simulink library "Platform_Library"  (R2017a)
settings: Solver=VariableStepAuto  StartTime=0.0  StopTime=10.0  RelTol=1e-3
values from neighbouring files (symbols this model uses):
  m = 0    [wavespec.m]
  n = 0    [wavespec.m]
  v_req_start = 14.5    [run_master.m]
  wpts = [32.8502 121.2880    [run_master.m]
undefined symbols (not defined in the file or in its folder): course_legs, course_legsBA, distnm_legs, distnm_legsBA, ship_cargo_capacity

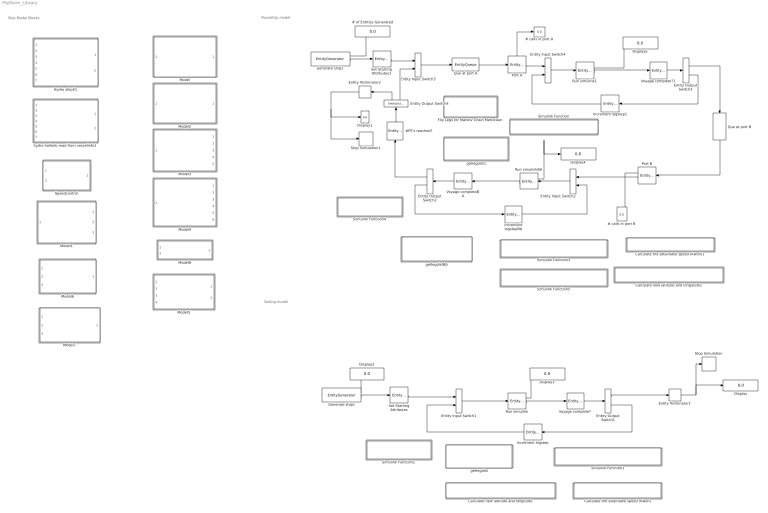
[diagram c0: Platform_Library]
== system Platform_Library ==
  note: Ship Model Blocks
  note: Roundtrip model
  note: Sailing model
  # calls in port A : Display
  # calls in port B : Display
  # of Entities Generated : Display
  #RT's reached? : EntityServer  InputPortMessageModes=m  OutputPortMessageModes=m  Capacity=1  ServiceTimeValue=0  EntryAction=|
      | %Add to the number of round trips (RTs) completed
      | entity.NumRTs=entity.NumRTs+1;
      | 
      | %Check to see if the desired number of RTs is reached
      | %If so, send entity to terminate simulation
      | entity.outputport=Completed_RT(entity.NumRTs);
  Calculate new latitude and longitude : Subsystem  TreatAsAtomicUnit=on
  Calculate new latitude and longitude1 : Subsystem  TreatAsAtomicUnit=on
  Calculate the attainable speed (Kwon) : Subsystem  TreatAsAtomicUnit=on
  Calculate the attainable speed (Kwon)1 : Subsystem  TreatAsAtomicUnit=on
  Display{,1..5} (6 alike) : Display
  Entity Input Switch{1..4} (4 alike) : EntityInputSwitch  InputPortMessageModes=m,m  OutputPortMessageModes=m
  Entity Output Switch{1..4} (4 alike) : EntityOutputSwitch  InputPortMessageModes=m  OutputPortMessageModes=m,m  SwitchingCriterion=From attribute  SwitchAttributeName=outputport
  Entity Terminator1 : EntityTerminator  InputPortMessageModes=m  NumberEntitiesArrived=on
  Entity Terminator2 : EntityTerminator  InputPortMessageModes=m  NumberEntitiesArrived=on
  Flip Legs for Markov Chain MetOcean : Subsystem  TreatAsAtomicUnit=on
  Generate ship1 : EntityGenerator  OutputPortMessageModes=n,m  TimeSource=MATLAB action  IntergenerationTimeAction=|  GenerateEntityAtSimulationStart=off  AttributeName=HsSea_S|HsdSea_S|TpSea_S|HsSwl_S|HsdSwl_S|TpSwl_S|u10_S|u10d_S|speed|outputport|legstep|legdist|leg|course|lat|lon|Hs4k|Hsd4k|Att_speed|Dist_sailed_tot|Dist_sailed_leg|numRTs|Voyage_step  AttributeInitialValue=0|0|0|0|0|0|0|0|15|1|2|1|1|1|1|1|1|1|1|0|0|1|1  NumberEntitiesDeparted=on  EntityType=Structured  EntityTypeName=ship
      | persistent count igt;
      | if isempty(count)
      |     igt=[0 inf];
      |     count=1;
      | end
      | dt=igt(count);
      | count=count+1;
  Generate ship2 : EntityGenerator  OutputPortMessageModes=n,m  TimeSource=MATLAB action  IntergenerationTimeAction=|  GenerateEntityAtSimulationStart=off  AttributeName=HsSea_S|HsdSea_S|TpSea_S|HsSwl_S|HsdSwl_S|TpSwl_S|u10_S|u10d_S|speed|outputport|legstep|legdist|leg|course|lat|lon|Hs4k|Hsd4k|Att_speed|Dist_sailed_tot|Dist_sailed_leg|NumRTs|Voyage_step|capacity  AttributeInitialValue=0|0|0|0|0|0|0|0|15|1|2|1|1|1|1|1|1|1|1|0|0|0|0|1  NumberEntitiesDeparted=on  EntityType=Structured  EntityTypeName=ship
      | persistent count igt;
      | if isempty(count)
      |     igt=[0 inf];
      |     count=1;
      | end
      | dt=igt(count);
      | count=count+1;
  Hydro shipX1 : ModelReference  ModelNameDialog=hydrodynamics.slx  SimulationMode=Normal  ModelReferenceVersion=1.29
  Increment legstep : EntityServer  InputPortMessageModes=m  OutputPortMessageModes=m  Capacity=1  ServiceTimeValue=0  EntryAction=|
      | %increment the total progress
      | entity.legstep=entity.legstep+1;
  Increment legstep1 : EntityServer  InputPortMessageModes=m  OutputPortMessageModes=m  Capacity=1  ServiceTimeValue=0  EntryAction=|
      | %increment the total progress
      | entity.legstep=entity.legstep+1;
  Increment legstepBA : EntityServer  InputPortMessageModes=m  OutputPortMessageModes=m  Capacity=1  ServiceTimeValue=0  EntryAction=|
      | %increment the total progress
      | entity.legstep=entity.legstep+1;
  Model : ModelReference  ModelNameDialog=EngRoomONE  SimulationMode=Normal  ModelReferenceVersion=1.56
  Model1 : ModelReference  ModelNameDialog=EngRoomBattery  SimulationMode=Normal  ModelReferenceVersion=1.71
  Model2 : ModelReference  ModelNameDialog=EngRoomTWO  SimulationMode=Normal  ModelReferenceVersion=1.51
  Model3 : ModelReference  ModelNameDialog=EngRoomTHREE  SimulationMode=Normal  ModelReferenceVersion=1.45
  Model4 : ModelReference  ModelNameDialog=EngRoomFOUR  SimulationMode=Normal  ModelReferenceVersion=1.44
  Model5 : ModelReference  ModelNameDialog=getLatLon  SimulationMode=Normal  ModelReferenceVersion=1.5
  Model6 : ModelReference  ModelNameDialog=Kwon_speed_loss  SimulationMode=Normal  ModelReferenceVersion=1.21
  Model7 : ModelReference  ModelNameDialog=Wind_Resistance_Model  SimulationMode=Normal  ModelReferenceVersion=1.5
  Model8 : ModelReference  ModelNameDialog=speedcontrol  SimulationMode=Normal  ModelReferenceVersion=1.22
  Port A : EntityServer  InputPortMessageModes=m  OutputPortMessageModes=n,m  Capacity=1  ServiceTimeValue=10  EntryAction=|  NumberEntitiesDeparted=on
      | %The ship is in port
      | 
      | %Run the ship model with the following modifications
      | %speed=0
      | %course=0
      | %Voyage_step: +0.5 (read as vessel being in port)
      | 
      | %run the ship model  and output the weather states (Markov Chain)
      | [HsSea_S,HsdSea_S,TpSea_S,HsSwl_S,HsdSwl_S,TpSwl_S,hsd4k,hs4k,u10_S,u10d_S]=runSim(entity.legstep, entity.course,entity.speed,entity.leg,...
      |                                                 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
  Port B : EntityServer  InputPortMessageModes=m  OutputPortMessageModes=n,m  Capacity=1  ServiceTimeValue=10  EntryAction=|  NumberEntitiesDeparted=on
      | %The ship is in port
      | 
      | %Run the ship model with the following modifications
      | %speed=0
      | %course=0
      | %Voyage_step: +0.5 (read as vessel being in port)
      | 
      | %run the ship model  and output the weather states (Markov Chain)
      | [HsSea_S,HsdSea_S,TpSea_S,HsSwl_S,HsdSwl_S,TpSwl_S,hsd4k,hs4k,u10_S,u10d_S]=runSim(entity.legstep, 0,0,entity.leg,...
      |                                                            entity.HsSwl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
  Que at port A : EntityQueue  InputPortMessageModes=m  OutputPortMessageModes=m
  Que at port B : EntityQueue  InputPortMessageModes=m  OutputPortMessageModes=m
  Run simulink : EntityServer  InputPortMessageModes=m  OutputPortMessageModes=n,m  Capacity=1  ServiceTimeValue=1  EntryAction=|  NumberEntitiesDeparted=on
      | %take the current leg, and give the vessel its course and the distance of the leg
      | [entity.course,entity.legdist]=readLeg(entity.leg);
      | 
      | %run the ship model, and output the weather states (Markov Chain)
      | [HsSea_S,HsdSea_S,TpSea_S,HsSwl_S,HsdSwl_S,TpSwl_S,hsd4k,hs4k,u10_S,u10d_S] = runSim(entity.legstep,entity.course,entity.speed,entity.leg,...
      |                                                    entity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
  Run simulink1 : EntityServer  InputPortMessageModes=m  OutputPortMessageModes=n,m  Capacity=1  ServiceTimeValue=1  EntryAction=|  NumberEntitiesDeparted=on
      | %take the current leg, and give the vessel its course and the distance of the leg
      | [entity.course,entity.legdist]=readLeg(entity.leg);
      | 
      | %run the ship model, and output the weather states (Markov Chain)
      | [HsSea_S,HsdSea_S,TpSea_S,HsSwl_S,HsdSwl_S,...
      |         TpSwl_S,hsd4k,hs4k,u10_S,u10d_S]  =  runSim(entity.legstep, entity.course,entity.speed,entity.leg,...
      |                                           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
  Run simulinkBA : EntityServer  InputPortMessageModes=m  OutputPortMessageModes=n,m  Capacity=1  ServiceTimeValue=1  EntryAction=|  NumberEntitiesDeparted=on
      | %take the current leg, and give the vessel its course and the distance of the leg
      | [entity.course,entity.legdist]=readLegBA(entity.leg); %reads from the flipped waypoints
      | 
      | %Flip leg number to collect the correct weather data for Markov Chain MetOcean
      | mc_leg=getmcleg(entity.leg);
      | 
      | %run the ship model, and output the weather states (Markov Chain)
      | [HsSea_S,HsdSea_S,TpSea_S,HsSwl_S,HsdSwl_S,...
      |        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
  Set Starting Attributes : EntityServer  InputPortMessageModes=m  OutputPortMessageModes=m  Capacity=1  ServiceTimeValue=0  EntryAction=|
      | %Read origin coordinates from waypoints
      | [lat1,lon1,v_req]=SetStart();
      | 
      | %Assign starting coordinates to entity
      | entity.lat=lat1;
      | entity.lon=lon1;
      | 
      | %Assign the intended speed
      | entity.speed=v_req;
  Set Starting Attributes1 : EntityServer  InputPortMessageModes=m  OutputPortMessageModes=m  Capacity=1  ServiceTimeValue=0  EntryAction=|
      | %Read origin coordinates from waypoints
      | [lat1,lon1,v_req,capacity]=SetStart();
      | 
      | %Assign starting coordinates to entity
      | entity.lat=lat1;
      | entity.lon=lon1;
      | 
      | %Assign the intended speed
      | entity.speed=v_req;
      | 
      | %Assign cargo capacity
      | entity.capacity=capacity;
  Simulink Function : Subsystem  TreatAsAtomicUnit=on
  Simulink Function1 : Subsystem  TreatAsAtomicUnit=on
  Simulink Function2 : Subsystem  TreatAsAtomicUnit=on
  Simulink Function3 : Subsystem  TreatAsAtomicUnit=on
  Simulink Function4 : Subsystem  TreatAsAtomicUnit=on
  Simulink Function5 : Subsystem  TreatAsAtomicUnit=on
  Speedcontrol : ModelReference  ModelNameDialog=speedcontrol.slx  SimulationMode=Normal  ModelReferenceVersion=1.22
  Stop Simulation : Stop
  Stop Simulation1 : Stop
  Voyage complete? : EntityServer  InputPortMessageModes=m  OutputPortMessageModes=m  Capacity=1  ServiceTimeValue=0  EntryAction=|
      | %Check if the entire voyage is complete
      | entity.outputport=checkComplete(entity.leg,entity.legdist,entity.Dist_sailed_leg);
      | 
      | %Check if the current Leg is complete
      | %if entity.Dist_sailed_leg>=entity.legdist
      |  %   entity.leg=entity.leg+1;%start new leg
      |  %   entity.legstep=1; %reset the counter to the new leg
      |   %  entity.Dist_sailed_leg=0; %reset the counter for distance sailed on current leg%
      | %end
  Voyage complete?1 : EntityServer  InputPortMessageModes=m  OutputPortMessageModes=m  Capacity=1  ServiceTimeValue=0  EntryAction=entity.outputport=checkComplete(entity.leg,entity.legdist,entity.Dist_sailed_leg);
  Voyage completeBA : EntityServer  InputPortMessageModes=m  OutputPortMessageModes=m  Capacity=1  ServiceTimeValue=0  EntryAction=entity.outputport=checkCompleteBA(entity.leg,entity.legdist,entity.Dist_sailed_leg);
  getlegdist : Subsystem  TreatAsAtomicUnit=on
  getlegdist1 : Subsystem  TreatAsAtomicUnit=on
  getlegdistBA : Subsystem  TreatAsAtomicUnit=on
  hydro hollenb read from vesselinfo1 : ModelReference  ModelNameDialog=hydroHollenbach  SimulationMode=Normal  ModelReferenceVersion=1.60
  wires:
  Entity Output Switch1/2 -> Increment legstep/1
  Entity Terminator1/1 -> Stop Simulation/1, Display/1
  Generate ship1/1 -> Display2/1
  Entity Output Switch1/1 -> Entity Terminator1/1
  Run simulink/2 -> Voyage complete?/1
  Set Starting Attributes/1 -> Entity Input Switch1/1
  Entity Input Switch1/1 -> Run simulink/1
  Generate ship1/2 -> Set Starting Attributes/1
  Voyage complete?/1 -> Entity Output Switch1/1
  Run simulink/1 -> Display3/1
  Increment legstep/1 -> Entity Input Switch1/2
  Que at port B/1 -> Port B/1
  Entity Input Switch2/1 -> Run simulinkBA/1
  Set Starting Attributes1/1 -> Entity Input Switch3/1
  Entity Input Switch4/1 -> Run simulink1/1
  Port B/2 -> Entity Input Switch2/1
  Run simulink1/2 -> Voyage complete?1/1
  Port B/1 -> # calls in port B/1
  Run simulinkBA/1 -> Display4/1
  Voyage complete?1/1 -> Entity Output Switch3/1
  Run simulink1/1 -> Display5/1
  Entity Terminator2/1 -> Stop Simulation1/1, Display1/1
  Increment legstepBA/1 -> Entity Input Switch2/2
  Entity Output Switch3/1 -> Que at port B/1
  #RT's reached?/1 -> Entity Output Switch4/1
  Port A/1 -> # calls in port A/1
  Generate ship2/1 -> # of Entities Generated/1
  Entity Output Switch2/1 -> #RT's reached?/1
  Entity Output Switch4/2 -> Entity Input Switch3/2
  Run simulinkBA/2 -> Voyage completeBA/1
  Entity Output Switch4/1 -> Entity Terminator2/1
  Entity Output Switch3/2 -> Increment legstep1/1
  Increment legstep1/1 -> Entity Input Switch4/2
  Voyage completeBA/1 -> Entity Output Switch2/1
  Que at port A/1 -> Port A/1
  Generate ship2/2 -> Set Starting Attributes1/1
  Entity Output Switch2/2 -> Increment legstepBA/1
  Entity Input Switch3/1 -> Que at port A/1
  Port A/2 -> Entity Input Switch4/1

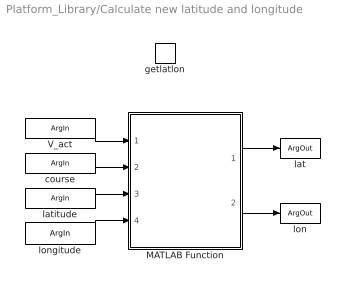
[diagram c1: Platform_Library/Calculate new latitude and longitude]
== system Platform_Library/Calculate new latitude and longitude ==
  getlatlon : TriggerPort  TriggerType=function-call  IsSimulinkFunction=on  FunctionName=getlatlon  VariantControl=Variant
  MATLAB Function : MATLAB Function  TreatAsAtomicUnit=on
  V_act : ArgIn  DisableCoverage=on  ArgumentName=V_act
  latitude : ArgIn  Port=2  ArgumentName=latitude
  longitude : ArgIn  Port=3  ArgumentName=longitude
  course : ArgIn  Port=4  ArgumentName=course
  lat : ArgOut  DisableCoverage=on  ArgumentName=lat
  lon : ArgOut  Port=2  ArgumentName=lon
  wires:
  V_act/1 -> MATLAB Function/1(V_act)
  MATLAB Function/1(lat_new) -> lat/1
  course/1 -> MATLAB Function/2(Course)
  latitude/1 -> MATLAB Function/3(Lat)
  longitude/1 -> MATLAB Function/4(Lon)
  MATLAB Function/2(lon_new) -> lon/1

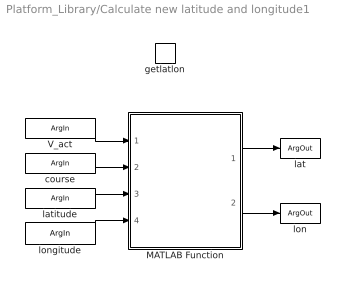
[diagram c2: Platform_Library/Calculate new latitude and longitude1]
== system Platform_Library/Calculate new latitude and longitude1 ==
  getlatlon : TriggerPort  TriggerType=function-call  IsSimulinkFunction=on  FunctionName=getlatlon  VariantControl=Variant
  MATLAB Function : MATLAB Function  TreatAsAtomicUnit=on
  V_act : ArgIn  DisableCoverage=on  ArgumentName=V_act
  latitude : ArgIn  Port=2  ArgumentName=latitude
  longitude : ArgIn  Port=3  ArgumentName=longitude
  course : ArgIn  Port=4  ArgumentName=course
  lat : ArgOut  DisableCoverage=on  ArgumentName=lat
  lon : ArgOut  Port=2  ArgumentName=lon
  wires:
  V_act/1 -> MATLAB Function/1(V_act)
  MATLAB Function/1(lat_new) -> lat/1
  course/1 -> MATLAB Function/2(Course)
  latitude/1 -> MATLAB Function/3(Lat)
  longitude/1 -> MATLAB Function/4(Lon)
  MATLAB Function/2(lon_new) -> lon/1

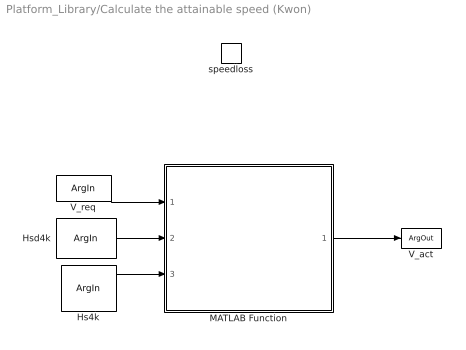
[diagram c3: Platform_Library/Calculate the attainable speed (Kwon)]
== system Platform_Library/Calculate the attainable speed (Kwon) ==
  speedloss : TriggerPort  TriggerType=function-call  IsSimulinkFunction=on  FunctionName=speedloss  VariantControl=Variant
  MATLAB Function : MATLAB Function  TreatAsAtomicUnit=on
  V_req : ArgIn  DisableCoverage=on  ArgumentName=V_req
  Hsd4k : ArgIn  Port=2  ArgumentName=Hsd4k
  Hs4k : ArgIn  Port=3  ArgumentName=Hs4k
  V_act : ArgOut  DisableCoverage=on  ArgumentName=V_act
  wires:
  MATLAB Function/1(V_act) -> V_act/1
  Hs4k/1 -> MATLAB Function/3(Hs)
  Hsd4k/1 -> MATLAB Function/2(rel_heading)
  V_req/1 -> MATLAB Function/1(V_req)

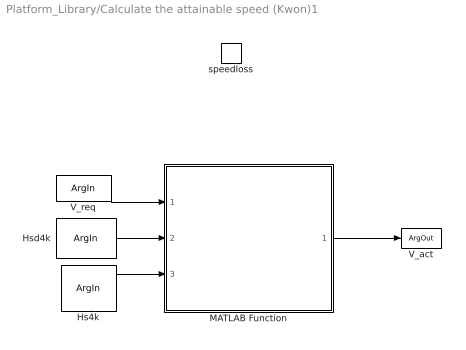
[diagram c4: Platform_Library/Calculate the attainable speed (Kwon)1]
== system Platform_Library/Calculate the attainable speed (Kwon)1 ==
  speedloss : TriggerPort  TriggerType=function-call  IsSimulinkFunction=on  FunctionName=speedloss  VariantControl=Variant
  MATLAB Function : MATLAB Function  TreatAsAtomicUnit=on
  V_req : ArgIn  DisableCoverage=on  ArgumentName=V_req
  Hsd4k : ArgIn  Port=2  ArgumentName=Hsd4k
  Hs4k : ArgIn  Port=3  ArgumentName=Hs4k
  V_act : ArgOut  DisableCoverage=on  ArgumentName=V_act
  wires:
  MATLAB Function/1(V_act) -> V_act/1
  Hs4k/1 -> MATLAB Function/3(Hs)
  Hsd4k/1 -> MATLAB Function/2(rel_heading)
  V_req/1 -> MATLAB Function/1(V_req)

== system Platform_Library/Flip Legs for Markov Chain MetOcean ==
  getmcleg : TriggerPort  TriggerType=function-call  IsSimulinkFunction=on  FunctionName=getmcleg  VariantControl=Variant
  MATLAB Function : MATLAB Function  TreatAsAtomicUnit=on
  leg : ArgIn  DisableCoverage=on  ArgumentName=leg
  mc_leg : ArgOut  DisableCoverage=on  ArgumentName=mc_leg
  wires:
  leg/1 -> MATLAB Function/1(leg)
  MATLAB Function/1(mc_leg) -> mc_leg/1

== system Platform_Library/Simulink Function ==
  Completed_RT : TriggerPort  TriggerType=function-call  IsSimulinkFunction=on  FunctionName=Completed_RT  VariantControl=Variant
  MATLAB Function : MATLAB Function  TreatAsAtomicUnit=on
  numRTs : ArgIn  DisableCoverage=on  ArgumentName=numRTs
  outputport : ArgOut  DisableCoverage=on  ArgumentName=outputport
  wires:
  numRTs/1 -> MATLAB Function/1(NumRTs)
  MATLAB Function/1(outport) -> outputport/1

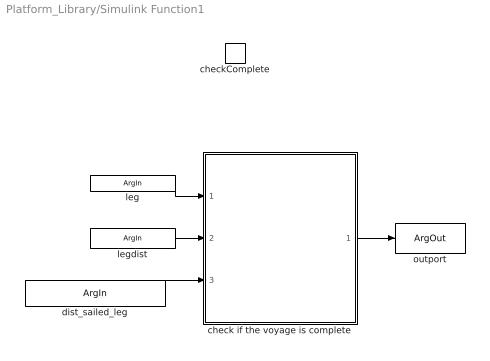
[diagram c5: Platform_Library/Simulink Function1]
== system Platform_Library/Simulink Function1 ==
  checkComplete : TriggerPort  TriggerType=function-call  IsSimulinkFunction=on  FunctionName=checkComplete  VariantControl=Variant
  check if the voyage is complete : MATLAB Function  TreatAsAtomicUnit=on
  leg : ArgIn  DisableCoverage=on  ArgumentName=leg
  legdist : ArgIn  Port=2  ArgumentName=legdist
  dist_sailed_leg : ArgIn  Port=3  ArgumentName=dist_sailed_leg
  outport : ArgOut  DisableCoverage=on  ArgumentName=outport
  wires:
  leg/1 -> check if the voyage is complete/1(leg)
  check if the voyage is complete/1(outport) -> outport/1
  dist_sailed_leg/1 -> check if the voyage is complete/3(dist_sailed_leg)
  legdist/1 -> check if the voyage is complete/2(legdist)

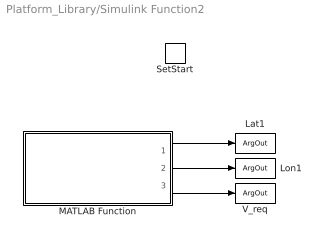
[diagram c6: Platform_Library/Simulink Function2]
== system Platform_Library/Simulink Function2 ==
  SetStart : TriggerPort  TriggerType=function-call  IsSimulinkFunction=on  FunctionName=SetStart  VariantControl=Variant
  MATLAB Function : MATLAB Function  TreatAsAtomicUnit=on
  Lat1 : ArgOut  DisableCoverage=on  ArgumentName=Lat1
  Lon1 : ArgOut  Port=2  ArgumentName=Lon1
  V_req : ArgOut  Port=3  ArgumentName=V_req
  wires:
  MATLAB Function/2(Lon1) -> Lon1/1
  MATLAB Function/1(Lat1) -> Lat1/1
  MATLAB Function/3(v_req) -> V_req/1

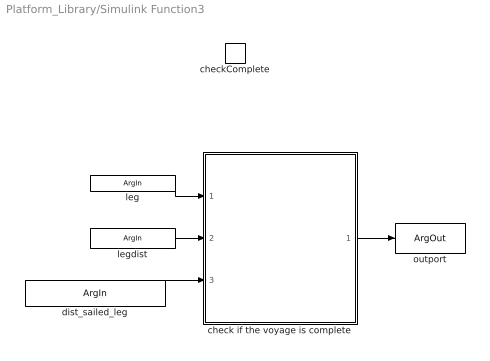
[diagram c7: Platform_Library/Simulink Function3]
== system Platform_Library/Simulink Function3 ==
  checkComplete : TriggerPort  TriggerType=function-call  IsSimulinkFunction=on  FunctionName=checkComplete  VariantControl=Variant
  check if the voyage is complete : MATLAB Function  TreatAsAtomicUnit=on
  leg : ArgIn  DisableCoverage=on  ArgumentName=leg
  legdist : ArgIn  Port=2  ArgumentName=legdist
  dist_sailed_leg : ArgIn  Port=3  ArgumentName=dist_sailed_leg
  outport : ArgOut  DisableCoverage=on  ArgumentName=outport
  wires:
  leg/1 -> check if the voyage is complete/1(leg)
  check if the voyage is complete/1(outport) -> outport/1
  dist_sailed_leg/1 -> check if the voyage is complete/3(dist_sailed_leg)
  legdist/1 -> check if the voyage is complete/2(legdist)

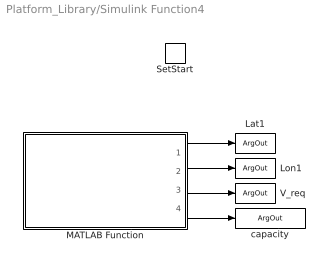
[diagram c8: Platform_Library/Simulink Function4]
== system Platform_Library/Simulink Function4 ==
  SetStart : TriggerPort  TriggerType=function-call  IsSimulinkFunction=on  FunctionName=SetStart  VariantControl=Variant
  MATLAB Function : MATLAB Function  TreatAsAtomicUnit=on
  Lat1 : ArgOut  DisableCoverage=on  ArgumentName=Lat1
  Lon1 : ArgOut  Port=2  ArgumentName=Lon1
  V_req : ArgOut  Port=3  ArgumentName=V_req
  capacity : ArgOut  Port=4  ArgumentName=capacity
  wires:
  MATLAB Function/2(Lon1) -> Lon1/1
  MATLAB Function/1(Lat1) -> Lat1/1
  MATLAB Function/3(v_req) -> V_req/1
  MATLAB Function/4(capacity) -> capacity/1

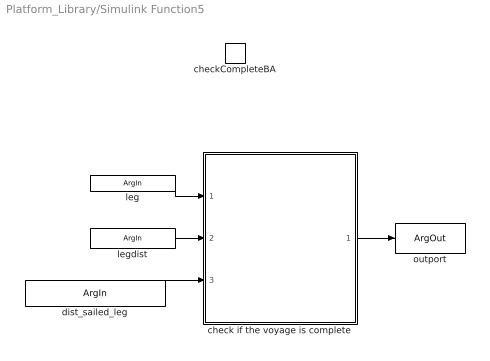
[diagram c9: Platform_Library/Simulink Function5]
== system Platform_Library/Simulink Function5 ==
  checkCompleteBA : TriggerPort  TriggerType=function-call  IsSimulinkFunction=on  FunctionName=checkCompleteBA  VariantControl=Variant
  check if the voyage is complete : MATLAB Function  TreatAsAtomicUnit=on
  leg : ArgIn  DisableCoverage=on  ArgumentName=leg
  legdist : ArgIn  Port=2  ArgumentName=legdist
  dist_sailed_leg : ArgIn  Port=3  ArgumentName=dist_sailed_leg
  outport : ArgOut  DisableCoverage=on  ArgumentName=outport
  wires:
  leg/1 -> check if the voyage is complete/1(leg)
  check if the voyage is complete/1(outport) -> outport/1
  dist_sailed_leg/1 -> check if the voyage is complete/3(dist_sailed_leg)
  legdist/1 -> check if the voyage is complete/2(legdist)

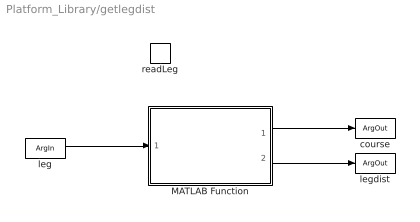
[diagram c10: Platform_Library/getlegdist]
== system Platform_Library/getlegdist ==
  readLeg : TriggerPort  TriggerType=function-call  IsSimulinkFunction=on  FunctionName=readLeg  VariantControl=Variant
  MATLAB Function : MATLAB Function  TreatAsAtomicUnit=on
  leg : ArgIn  DisableCoverage=on  ArgumentName=leg
  course : ArgOut  DisableCoverage=on  ArgumentName=course
  legdist : ArgOut  DisableCoverage=on  Port=2  ArgumentName=legdist
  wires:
  leg/1 -> MATLAB Function/1(leg)
  MATLAB Function/1(course) -> course/1
  MATLAB Function/2(legdist) -> legdist/1

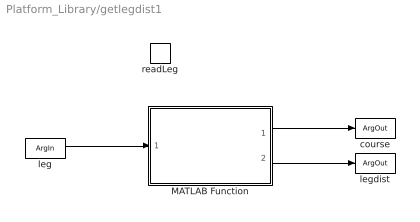
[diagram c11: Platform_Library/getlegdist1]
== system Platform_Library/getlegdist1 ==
  readLeg : TriggerPort  TriggerType=function-call  IsSimulinkFunction=on  FunctionName=readLeg  VariantControl=Variant
  MATLAB Function : MATLAB Function  TreatAsAtomicUnit=on
  leg : ArgIn  DisableCoverage=on  ArgumentName=leg
  course : ArgOut  DisableCoverage=on  ArgumentName=course
  legdist : ArgOut  DisableCoverage=on  Port=2  ArgumentName=legdist
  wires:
  leg/1 -> MATLAB Function/1(leg)
  MATLAB Function/1(course) -> course/1
  MATLAB Function/2(legdist) -> legdist/1

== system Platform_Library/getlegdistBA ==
  readLegBA : TriggerPort  TriggerType=function-call  IsSimulinkFunction=on  FunctionName=readLegBA  VariantControl=Variant
  MATLAB Function : MATLAB Function  TreatAsAtomicUnit=on
  leg : ArgIn  DisableCoverage=on  ArgumentName=leg
  course : ArgOut  DisableCoverage=on  ArgumentName=course
  legdist : ArgOut  DisableCoverage=on  Port=2  ArgumentName=legdist
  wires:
  leg/1 -> MATLAB Function/1(leg)
  MATLAB Function/1(course) -> course/1
  MATLAB Function/2(legdist) -> legdist/1

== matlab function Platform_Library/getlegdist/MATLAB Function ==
function [course,legdist] = fcn(leg,distnm_legs,course_legs)
%take in the current leg that the vessel is on, and give the distance for
%that leg, and the course
course=course_legs(leg);
legdist=distnm_legs(leg);
    
end

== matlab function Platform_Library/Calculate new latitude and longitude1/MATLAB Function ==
function [lat_new, lon_new] = New_Lat_Lon(V_act,Course,Lat,Lon)

coder.extrinsic('nm2deg')
coder.extrinsic('reckon')
time=1; % one hour time steps

lat_new=0; %preallocate
lon_new=0; %preallocate


distance=V_act*time; %distance sailed [nm]
arc_length=nm2deg(distance); %distance sailed [deg]

[lat_new, lon_new]=reckon(Lat,Lon,arc_length,Course); %new lat and lon


end

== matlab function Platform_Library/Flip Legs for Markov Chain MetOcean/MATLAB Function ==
function mc_leg = getMCleg(leg,distnm_legsBA)

%Flip the leg number to collect the correct weather data for MetOcean
%Markov Chains

num_legs=size(distnm_legsBA,1); %get the total number of legs
legs=(1:1:num_legs);
flip_legs=flip(legs);
mc_leg=flip_legs(leg);
end

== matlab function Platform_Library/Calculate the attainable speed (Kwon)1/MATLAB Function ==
function V_act = speedloss_Kwon(V_req,rel_heading,Hs, num)
coder.extrinsic('wrapTo180')
%Use Kwons method to estimate the speed loss due to added resistance

%pre allocate values
V_act=0;
V_2=0; %pre allocate the new speed
Bn=0;
Volume_deplacement=0;
C_u=0;
C_beta=0;
C_form=0;
heading_rel=0;

V_1=V_req*0.5144; %Convert the required speed (set speed) from kts to m/s
heading_rel=abs(wrapTo180(rel_heading)); %convert to 0-180 degrees
Volume_deplacement=num(54); %[m^3]
L=num(3); %Use Lwl
C_B=num(8); %block Coefficient



%calculate the current Froude Number
F_n=V_1/((9.81*L)^0.5);

%Get Beaufort scale number from waveheight
if Hs<0.2
    Bn=1;
elseif Hs>=0.2 && Hs<0.5
    Bn=2;
elseif Hs>=0.5 && Hs<1
    Bn=3;
elseif Hs>=1 && Hs<2
    Bn=4;
elseif Hs>2 && Hs<3
    Bn=5;
elseif Hs>3 && Hs<4
    Bn=6;
elseif Hs>4 %&& Hs<5.5
    Bn=7;
else
    disp('Bn is too high for Kwons method')
end
    

%calculate speed reduction coefficient
if C_B>=0.55 && C_B<0.575
    C_u=1.7-(1.4*F_n)-(7.4*(F_n^2));
elseif C_B>=0.575 && C_B<0.625
    C_u=2.2-(2.5*F_n)-(9.7*(F_n^2));
elseif C_B>=0.625 && C_B<0.675
    C_u=2.6-(3.7*F_n)-(11.6*(F_n^2));
elseif C_B>=0.675 && C_B<0.725
    C_u=3.1-(5.3*F_n)-(12.4*(F_n^2));
elseif C_B>=0.725 && C_B<0.775
    C_u=2.4-(10.6*F_n)-(9.5*(F_n^2));
elseif C_B>=0.775 && C_B<0.825
    C_u=2.6-(13.1*F_n)-(15.1*(F_n^2));
else %C_B>=0.825
    C_u=3.1-(18.7*F_n)+(28*(F_n^2));
end

%calculate direction reduction coefficient
if heading_rel>=0 && heading_rel<30 %head sea
    C_beta=1;
elseif heading_rel>=30 && heading_rel<60 %Bow sea
    C_beta=(1.7-0.03*((Bn-4)^2))/2;
elseif heading_rel>=60 && heading_rel<150 %Beam sea
    C_beta=(0.9-0.06*((Bn-6)^2))/2;
else %heading_rel>=150 && heading_rel<180 %Following sea
    C_beta=(0.4-0.03*((Bn-8)^2))/2;
end

%calculate the ship form coefficient
%valid for all ships, exept container ships, in loaded condition
%C_form=(0.5*Bn)+((Bn^(6.5))/((2.7*(Volume_deplacement^(2/3)))));

%valid for container ships in normal condition
C_form=(0.7*Bn)+((Bn^(6.5))/((22*(Volume_deplacement^(2/3)))));

%percentage loss calculated
%percentage_loss=((V_1-V_2)/V_1)*100;





%calculate deltaV/V1*100%
%Delta_V_overV=C_beta*C_u*C_form;
%coefficient=C_form*C_beta*C_u
%calculate actual ship speed in the selected weather [m/s]
% V_2=V_1-((Delta_V_overV)*(V_1/100))
V_2=V_1-((C_beta*C_u*C_form)*(V_1/100));

%calculate the absolute speed loss [m/s]
%delta_V=V_1-V_2



%if the speed loss found is negative, set the speed to the original speed
% This means that the approximate method did not work in this case
% if V_2>=V_1
%     V_2=V_1; 
%     disp('Approximate method not valid')
%     
% end

V_act=V_2/0.5144; % The actual attainable speed in kts
end


% %function V_act = speedloss_Kwon(V_req,rel_heading,Hs, num)
% %Use Kwons method to estimate the speed loss due to added resistance
% 
% V_1=V_req*0.5144; %Convert the required speed (set speed) from kts to m/s
% heading_rel=rel_heading;
% Volume_deplacement=num(54); %[m^3]
% L=num(3); %Use Lwl
% C_B=num(8); %block Coefficient
% 
% 
% %calculate the current Froude Number
% F_n=V_1/((9.81*L)^0.5);
% 
% %Get Beaufort scale number from waveheight
% if Hs<0.2
%     Bn=1;
% elseif Hs>=0.2 && Hs<0.5
%     Bn=2;
% elseif Hs>=0.5 && Hs<1
%     Bn=3;
% elseif Hs>=1 && Hs<2
%     Bn=4;
% elseif Hs>2 && Hs<3
%     Bn=5;
% elseif Hs>3 && Hs<4
%     Bn=6;
% elseif Hs>4 && Hs<5.5
%     Bn=7;
% else
%     disp('Bn is too high for Kwons method')
% end
%     
% 
% %calculate speed reduction coefficient
% if C_B>=0.55 && C_B<0.575
%     C_u=1.7-(1.4*F_n)-(7.4*(F_n^2));
% elseif C_B>=0.575 && C_B<0.625
%     C_u=2.2-(2.5*F_n)-(9.7*(F_n^2));
% elseif C_B>=0.625 && C_B<0.675
%     C_u=2.6-(3.7*F_n)-(11.6*(F_n^2));
% elseif C_B>=0.675 && C_B<0.725
%     C_u=3.1-(5.3*F_n)-(12.4*(F_n^2));
% elseif C_B>=0.725 && C_B<0.775
%     C_u=2.4-(10.6*F_n)-(9.5*(F_n^2));
% elseif C_B>=0.775 && C_B<0.825
%     C_u=2.6-(13.1*F_n)-(15.1*(F_n^2));
% elseif C_B>=0.825
%     C_u=3.1-(18.7*F_n)+(28*(F_n^2));
% end
% 
% %calculate direction reduction coefficient
% if heading_rel>=0 && heading_rel<30 %head sea
%     C_beta=1;
% elseif heading_rel>=30 && heading_rel<60 %Bow sea
%     C_beta=(1.7-0.03*((Bn-4)^2))/2;
% elseif heading_rel>=60 && heading_rel<150 %Beam sea
%     C_beta=(0.9-0.06*((Bn-6)^2))/2;
% elseif heading_rel>=150 && heading_rel<180 %Following sea
%     C_beta=(0.4-0.03*((Bn-8)^2))/2;
% end
% 
% %calculate the ship form coefficient
% %valid for all ships, exept container ships, in loaded condition
% C_form=(0.5*Bn)+((Bn^(6.5))/((2.7*(Volume_deplacement^(2/3)))));
% 
% %calculate deltaV/V1*100%
% %Delta_V_overV=C_beta*C_u*C_form;
% 
% %calculate actual ship speed in the selected weather [m/s]
% % V_2=V_1-((Delta_V_overV)*(V_1/100))
% V_2=V_1-((C_beta*C_u*C_form)*(V_1/100));
% 
% %calculate the absolute speed loss [m/s]
% %delta_V=V_1-V_2
% 
% %percentage loss calculated
% %percentage_loss=((V_1-V_2)/V_1)*100;
% 
% %if the speed loss found is negative, set the speed to the original speed
% % This means that the approximate method did not work in this case
% if V_2>=V_1
%     V_2=V_1; 
%     disp('Approximate method not valid')
%     
% end
% 
% V_act=V_2/0.5144; % The actual attainable speed in kts
% 
% end

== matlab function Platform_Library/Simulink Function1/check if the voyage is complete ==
function outport = fcn(leg,legdist,dist_sailed_leg,distnm_legs)

dist=dist_sailed_leg; %the distance sailed on current leg

if leg == length(distnm_legs) && dist>=(legdist-20) %subtract to avoid errors
    outport=1; %Journey complete
else
    outport=2; %Journey not complete
end

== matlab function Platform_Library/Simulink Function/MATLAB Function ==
function outport = outputportRT(NumRTs,SetNumRTs)



if NumRTs>=SetNumRTs
outport = 1; %Simulation is complete, end simulation
else
    outport=2; %Simulation is not complete, do another roundtrip
end
end

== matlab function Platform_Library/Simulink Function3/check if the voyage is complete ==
function outport = fcn(leg,legdist,dist_sailed_leg,distnm_legs)

dist=dist_sailed_leg; %the distance sailed on current leg

if leg == length(distnm_legs) && dist>=(legdist-20) %subtract to avoid errors
    outport=1; %Journey complete
else
    outport=2; %Journey not complete
end

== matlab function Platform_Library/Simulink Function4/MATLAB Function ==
function [Lat1, Lon1, v_req, capacity]= SetStartAttributes(wpts,v_req_start,ship_cargo_capacity)

start=zeros(1,2);
v_req=0;

start(1,1)=wpts(1,1); %Starting Latitude
start(1,2)=wpts(1,2); %Starting Longitute

Lat1=start(1,1);
Lon1=start(1,2);

v_req=v_req_start;

capacity=ship_cargo_capacity;
end

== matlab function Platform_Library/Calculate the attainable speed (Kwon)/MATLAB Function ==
function V_act = speedloss_Kwon(V_req,rel_heading,Hs, num)
coder.extrinsic('wrapTo180')
%Use Kwons method to estimate the speed loss due to added resistance

%pre allocate values
V_act=0;
V_2=0; %pre allocate the new speed
Bn=0;
Volume_deplacement=0;
C_u=0;
C_beta=0;
C_form=0;
heading_rel=0;

V_1=V_req*0.5144; %Convert the required speed (set speed) from kts to m/s
heading_rel=abs(wrapTo180(rel_heading)); %convert to 0-180 degrees
Volume_deplacement=num(54); %[m^3]
L=num(3); %Use Lwl
C_B=num(8); %block Coefficient



%calculate the current Froude Number
F_n=V_1/((9.81*L)^0.5);

%Get Beaufort scale number from waveheight
if Hs<0.2
    Bn=1;
elseif Hs>=0.2 && Hs<0.5
    Bn=2;
elseif Hs>=0.5 && Hs<1
    Bn=3;
elseif Hs>=1 && Hs<2
    Bn=4;
elseif Hs>2 && Hs<3
    Bn=5;
elseif Hs>3 && Hs<4
    Bn=6;
elseif Hs>4 %&& Hs<5.5
    Bn=7;
else
    disp('Bn is too high for Kwons method')
end
    

%calculate speed reduction coefficient
if C_B>=0.55 && C_B<0.575
    C_u=1.7-(1.4*F_n)-(7.4*(F_n^2));
elseif C_B>=0.575 && C_B<0.625
    C_u=2.2-(2.5*F_n)-(9.7*(F_n^2));
elseif C_B>=0.625 && C_B<0.675
    C_u=2.6-(3.7*F_n)-(11.6*(F_n^2));
elseif C_B>=0.675 && C_B<0.725
    C_u=3.1-(5.3*F_n)-(12.4*(F_n^2));
elseif C_B>=0.725 && C_B<0.775
    C_u=2.4-(10.6*F_n)-(9.5*(F_n^2));
elseif C_B>=0.775 && C_B<0.825
    C_u=2.6-(13.1*F_n)-(15.1*(F_n^2));
else %C_B>=0.825
    C_u=3.1-(18.7*F_n)+(28*(F_n^2));
end

%calculate direction reduction coefficient
if heading_rel>=0 && heading_rel<30 %head sea
    C_beta=1;
elseif heading_rel>=30 && heading_rel<60 %Bow sea
    C_beta=(1.7-0.03*((Bn-4)^2))/2;
elseif heading_rel>=60 && heading_rel<150 %Beam sea
    C_beta=(0.9-0.06*((Bn-6)^2))/2;
else %heading_rel>=150 && heading_rel<180 %Following sea
    C_beta=(0.4-0.03*((Bn-8)^2))/2;
end

%calculate the ship form coefficient
%valid for all ships, exept container ships, in loaded condition
%C_form=(0.5*Bn)+((Bn^(6.5))/((2.7*(Volume_deplacement^(2/3)))));

%valid for container ships in normal condition
C_form=(0.7*Bn)+((Bn^(6.5))/((22*(Volume_deplacement^(2/3)))));

%percentage loss calculated
%percentage_loss=((V_1-V_2)/V_1)*100;





%calculate deltaV/V1*100%
%Delta_V_overV=C_beta*C_u*C_form;
%coefficient=C_form*C_beta*C_u
%calculate actual ship speed in the selected weather [m/s]
% V_2=V_1-((Delta_V_overV)*(V_1/100))
V_2=V_1-((C_beta*C_u*C_form)*(V_1/100));

%calculate the absolute speed loss [m/s]
%delta_V=V_1-V_2



%if the speed loss found is negative, set the speed to the original speed
% This means that the approximate method did not work in this case
% if V_2>=V_1
%     V_2=V_1; 
%     disp('Approximate method not valid')
%     
% end

V_act=V_2/0.5144; % The actual attainable speed in kts
end


% %function V_act = speedloss_Kwon(V_req,rel_heading,Hs, num)
% %Use Kwons method to estimate the speed loss due to added resistance
% 
% V_1=V_req*0.5144; %Convert the required speed (set speed) from kts to m/s
% heading_rel=rel_heading;
% Volume_deplacement=num(54); %[m^3]
% L=num(3); %Use Lwl
% C_B=num(8); %block Coefficient
% 
% 
% %calculate the current Froude Number
% F_n=V_1/((9.81*L)^0.5);
% 
% %Get Beaufort scale number from waveheight
% if Hs<0.2
%     Bn=1;
% elseif Hs>=0.2 && Hs<0.5
%     Bn=2;
% elseif Hs>=0.5 && Hs<1
%     Bn=3;
% elseif Hs>=1 && Hs<2
%     Bn=4;
% elseif Hs>2 && Hs<3
%     Bn=5;
% elseif Hs>3 && Hs<4
%     Bn=6;
% elseif Hs>4 && Hs<5.5
%     Bn=7;
% else
%     disp('Bn is too high for Kwons method')
% end
%     
% 
% %calculate speed reduction coefficient
% if C_B>=0.55 && C_B<0.575
%     C_u=1.7-(1.4*F_n)-(7.4*(F_n^2));
% elseif C_B>=0.575 && C_B<0.625
%     C_u=2.2-(2.5*F_n)-(9.7*(F_n^2));
% elseif C_B>=0.625 && C_B<0.675
%     C_u=2.6-(3.7*F_n)-(11.6*(F_n^2));
% elseif C_B>=0.675 && C_B<0.725
%     C_u=3.1-(5.3*F_n)-(12.4*(F_n^2));
% elseif C_B>=0.725 && C_B<0.775
%     C_u=2.4-(10.6*F_n)-(9.5*(F_n^2));
% elseif C_B>=0.775 && C_B<0.825
%     C_u=2.6-(13.1*F_n)-(15.1*(F_n^2));
% elseif C_B>=0.825
%     C_u=3.1-(18.7*F_n)+(28*(F_n^2));
% end
% 
% %calculate direction reduction coefficient
% if heading_rel>=0 && heading_rel<30 %head sea
%     C_beta=1;
% elseif heading_rel>=30 && heading_rel<60 %Bow sea
%     C_beta=(1.7-0.03*((Bn-4)^2))/2;
% elseif heading_rel>=60 && heading_rel<150 %Beam sea
%     C_beta=(0.9-0.06*((Bn-6)^2))/2;
% elseif heading_rel>=150 && heading_rel<180 %Following sea
%     C_beta=(0.4-0.03*((Bn-8)^2))/2;
% end
% 
% %calculate the ship form coefficient
% %valid for all ships, exept container ships, in loaded condition
% C_form=(0.5*Bn)+((Bn^(6.5))/((2.7*(Volume_deplacement^(2/3)))));
% 
% %calculate deltaV/V1*100%
% %Delta_V_overV=C_beta*C_u*C_form;
% 
% %calculate actual ship speed in the selected weather [m/s]
% % V_2=V_1-((Delta_V_overV)*(V_1/100))
% V_2=V_1-((C_beta*C_u*C_form)*(V_1/100));
% 
% %calculate the absolute speed loss [m/s]
% %delta_V=V_1-V_2
% 
% %percentage loss calculated
% %percentage_loss=((V_1-V_2)/V_1)*100;
% 
% %if the speed loss found is negative, set the speed to the original speed
% % This means that the approximate method did not work in this case
% if V_2>=V_1
%     V_2=V_1; 
%     disp('Approximate method not valid')
%     
% end
% 
% V_act=V_2/0.5144; % The actual attainable speed in kts
% 
% end

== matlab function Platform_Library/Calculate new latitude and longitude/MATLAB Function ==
function [lat_new, lon_new] = New_Lat_Lon(V_act,Course,Lat,Lon)

coder.extrinsic('nm2deg')
coder.extrinsic('reckon')
time=1; % one hour time steps

lat_new=0; %preallocate
lon_new=0; %preallocate


distance=V_act*time; %distance sailed [nm]
arc_length=nm2deg(distance); %distance sailed [deg]

[lat_new, lon_new]=reckon(Lat,Lon,arc_length,Course); %new lat and lon


end

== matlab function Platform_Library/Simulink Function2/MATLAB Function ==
function [Lat1, Lon1, v_req]= SetStartAttributes(wpts,v_req_start)

start=zeros(1,2);
v_req=0;

start(1,1)=wpts(1,1); %Starting Latitude
start(1,2)=wpts(1,2); %Starting Longitute

Lat1=start(1,1);
Lon1=start(1,2);

v_req=v_req_start;
end

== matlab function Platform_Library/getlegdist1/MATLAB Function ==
function [course,legdist] = fcn(leg,distnm_legs,course_legs)
%take in the current leg that the vessel is on, and give the distance for
%that leg, and the course
course=course_legs(leg);
legdist=distnm_legs(leg);
    
end

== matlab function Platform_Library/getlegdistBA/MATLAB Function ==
function [course,legdist] = fcn(leg,distnm_legsBA,course_legsBA)
%take in the current leg that the vessel is on, and give the distance for
%that leg, and the course
course = course_legsBA(leg);
legdist = distnm_legsBA(leg);
    
end

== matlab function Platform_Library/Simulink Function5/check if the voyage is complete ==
function outport = fcn(leg,legdist,dist_sailed_leg,distnm_legs)

dist=dist_sailed_leg; %the distance sailed on current leg

if leg == length(distnm_legs) && dist>=(legdist-20) %subtract to avoid errors
    outport=1; %Journey complete
else
    outport=2; %Journey not complete
end
